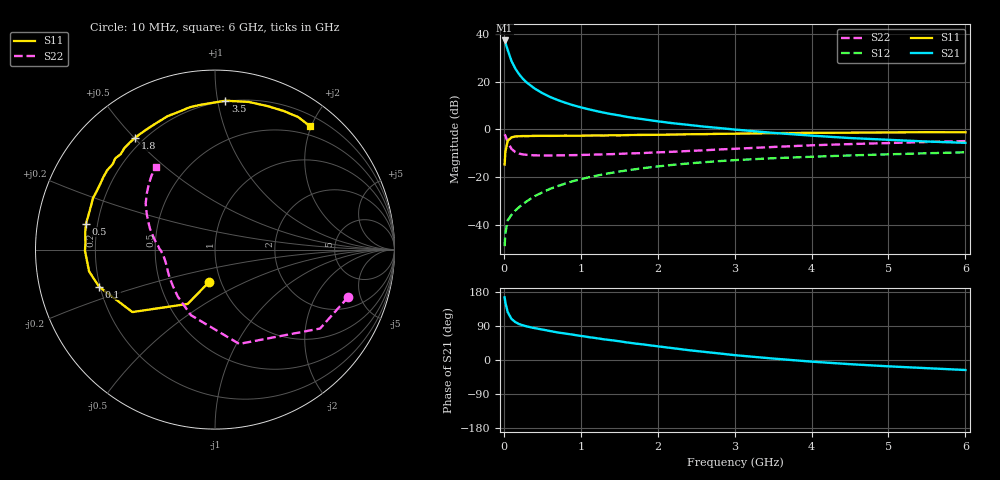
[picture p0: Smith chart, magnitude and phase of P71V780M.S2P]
! SIEMENS Small Signal Semiconductors
! BFP196
! Si NPN RF Bipolar Junction Transistor in SOT143
! VCE = 1.75 V  IC = 80 mA
! Common Emitter S-Parameters:  May  1996
# GHz  S  MA  R  50
!  f  S11  S21  S12  S22
! GHz  MAG  ANG  MAG  ANG  MAG  ANG  MAG  ANG
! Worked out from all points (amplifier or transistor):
!   36 points, 10 MHz to 6 GHz, reference 50 ohm
!   highest |S21| = 37.2 dB at 10 MHz (marker M1)
!   |S21| within 3 dB of that: start of sweep to 40.57 MHz
!   unconditionally stable (mu >= 1): 294.1 MHz to 5.144 GHz; 5.764 GHz to end of sweep
!   at 250 MHz: K = 0.95, MSG = 26.1 dB, |S12| = -31.2 dB
!   at 1.4 GHz: K = 1.10, MAG = 10.4 dB, |S12| = -18.2 dB
!   at 6 GHz: K = 1.01, MAG = 1.4 dB, |S12| = -9.6 dB
!   S11 on the Smith chart (normalised r, x): 10 MHz: 0.88, -0.33; 100 MHz: 0.20, -0.15; 500 MHz: 0.16, +0.10; 1.8 GHz: 0.17, +0.50; 3.5 GHz: 0.20, +1.05; 6 GHz: 0.36, +1.98
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0.01  0.1843 -100.4  72.35 165.5  0.0036 74.9  0.7883 -19.5
0.02  0.3388 -116.7  65.69 151.8  0.0067 63.1  0.7323 -36.9
0.05  0.5769 -142.9  45.7 126.4  0.0125 52.0  0.5424 -75.6
0.1  0.6785 -162.3  26.8 108.3  0.0163 51.5  0.3893 -110.1
0.15  0.712 -170.2  18.57 99.9  0.0201 53.7  0.334 -128.3
0.2  0.7167 -175.5  14.12 94.7  0.0237 57.4  0.3101 -139.2
0.25  0.7245 -179.5  11.31 91.3  0.0276 60.3  0.2984 -147.1
0.3  0.7227 177.5  9.463 88.5  0.0314 62.5  0.2928 -151.9
0.4  0.7295 172.2  7.151 84.1  0.04 64.6  0.2859 -159.1
0.5  0.733 168.6  5.73 80.4  0.0479 66.1  0.2839 -163.7
0.6  0.7307 164.5  4.771 76.5  0.0569 66.3  0.2841 -166.8
0.7  0.7327 160.4  4.103 72.7  0.0649 66.0  0.2857 -169.3
0.9  0.7351 153.9  3.2 66.7  0.0826 64.0  0.2887 -173.0
1.1  0.7413 147.3  2.635 60.5  0.0989 61.9  0.2941 -175.7
1.4  0.753 137.6  2.077 52.2  0.1231 57.6  0.3032 -179.3
1.8  0.7655 125.5  1.639 41.4  0.1534 51.6  0.3187 176.1
2.2  0.7767 115.1  1.341 31.1  0.181 45.3  0.3398 170.9
2.8  0.8059 99.9  1.066 17.3  0.2163 36.1  0.3794 162.4
3.5  0.8317 86.0  0.844 3.8  0.2487 25.8  0.4278 152.7
4.5  0.8515 69.8  0.658 -11.0  0.2848 13.6  0.4918 140.6
5.5  0.8721 57.8  0.556 -21.6  0.3162 2.8  0.5439 130.5
6  0.8672 52.5  0.522 -26.4  0.3311 -3.0  0.5681 125.5
